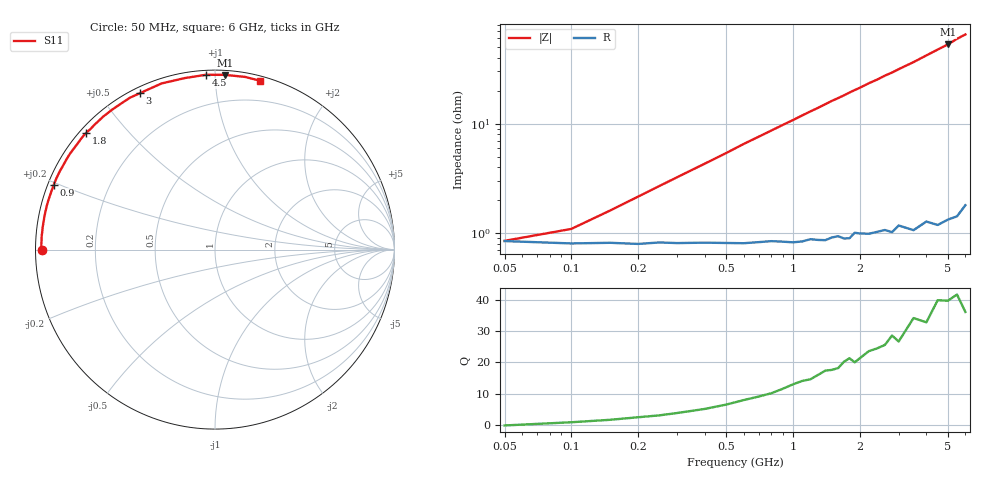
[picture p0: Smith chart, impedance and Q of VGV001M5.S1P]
! Infineon Technologies  Discrete & RF Semiconductors
! BB 831
! Si Tuning Diode in SOD323
! VR =
! S-Parameters:  July  1999
# GHz  S  MA  R  50
!  f  S11
! GHz  MAG  ANG
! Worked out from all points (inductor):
!   34 points, 50 MHz to 6 GHz, reference 50 ohm
!   read as one part to ground: L = 1.67 nH near 250 MHz
!   highest Q = 39.8 at 5 GHz (marker M1), where L = 1.68 nH
!   S11 on the Smith chart (normalised r, x): 50 MHz: 0.02, -0.00; 900 MHz: 0.02, +0.19; 1.8 GHz: 0.02, +0.38; 3 GHz: 0.02, +0.63; 4.5 GHz: 0.02, +0.95; 6 GHz: 0.04, +1.30
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0.05  0.9666 -179.8
0.1  0.9681 178.3
0.2  0.9685 175.4
0.3  0.968 172.8
0.5  0.9682 167.8
0.6  0.9685 165.2
0.8  0.9676 160.4
0.9  0.9681 158.0
1  0.9688 155.7
1.2  0.9674 151.0
1.4  0.9687 146.5
1.5  0.9673 144.2
1.6  0.9668 142.2
1.7  0.9688 140.1
1.8  0.969 137.9
1.9  0.9658 135.9
2  0.9667 134.0
2.2  0.968 129.9
2.4  0.9676 126.4
2.6  0.9675 122.5
2.8  0.9699 119.3
3  0.9667 115.7
3.5  0.9725 107.8
4  0.9704 100.0
4.5  0.9752 93.0
5  0.9751 86.8
5.5  0.9766 80.1
6  0.9736 75.0
